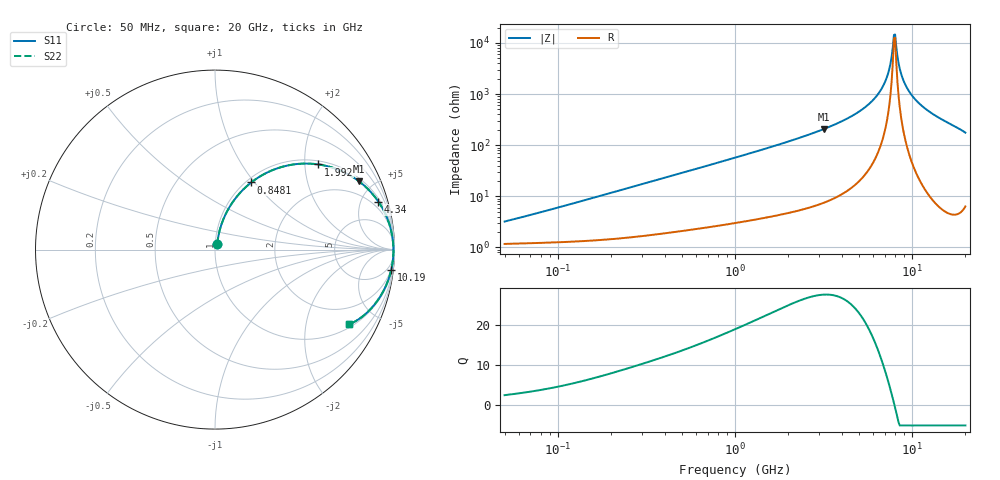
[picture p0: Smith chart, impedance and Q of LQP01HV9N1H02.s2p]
!Murata Part Number: LQP01HV9N1H02
!These Parameters are Measured in Series Mode Connection
!  o--[Z]--o
!Port1  Port2
!  o-------o
!Freq. Start=50[MHz] Stop=20[GHz], 401[Steps]
# Hz S RI R 50
!Freq.(Hz) S11(Real) S11(Imag) S21(Real) S21(Imag) S12(Real) S12(Imag) S22(Real) S22(Imag)
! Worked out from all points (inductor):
!   401 points, 50 MHz to 20 GHz, reference 50 ohm
!   read as one part in series: L = 9.43 nH near 60.75 MHz
!   highest Q = 27.6 at 3.169 GHz (marker M1), where L = 10.4 nH
!   self-resonance near 7.902 GHz
!   S11 on the Smith chart (normalised r, x): 50 MHz: 1.02, +0.06; 848.1 MHz: 1.05, +0.96; 1.992 GHz: 1.09, +2.35; 4.34 GHz: 1.26, +6.74; 10.19 GHz: 2, -17; 20 GHz: 1.13, -3.52
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5e7  0.0125 0.0292  0.9875 -0.0292  0.9875 -0.0292  0.0125 0.0292
1.364002e8  0.0192 0.0774  0.9808 -0.0774  0.9808 -0.0774  0.0192 0.0774
3.721004e8  0.0595 0.1977  0.9405 -0.1977  0.9405 -0.1977  0.0595 0.1977
8.480927e8  0.2023 0.3744  0.7977 -0.3744  0.7977 -0.3744  0.2023 0.3744
1e9  0.256 0.4109  0.744 -0.4109  0.744 -0.4109  0.256 0.4109
1.99176e9  0.5766 0.4745  0.4234 -0.4745  0.4234 -0.4745  0.5766 0.4745
2.728004e9  0.7352 0.4232  0.2648 -0.4232  0.2648 -0.4232  0.7352 0.4232
3.168813e9  0.8016 0.3811  0.1984 -0.3811  0.1984 -0.3811  0.8016 0.3811
4.34015e9  0.9106 0.2667  0.0894 -0.2667  0.0894 -0.2667  0.9106 0.2667
5.352748e9  0.958 0.1783  0.042 -0.1783  0.042 -0.1783  0.958 0.1783
6.217679e9  0.9797 0.1121  0.0203 -0.1121  0.0203 -0.1121  0.9797 0.1121
6.905011e9  0.989 0.0649  0.011 -0.0649  0.011 -0.0649  0.989 0.0649
7.442007e9  0.9928 0.0309  0.00723 -0.0309  0.00723 -0.0309  0.9928 0.0309
7.784049e9  0.9939 0.0104  0.00614 -0.0104  0.00614 -0.0104  0.9939 0.0104
8.020766e9  0.9941 -0.00335  0.0059 0.00335  0.0059 0.00335  0.9941 -0.00335
8.141811e9  0.9941 -0.0102  0.00593 0.0102  0.00593 0.0102  0.9941 -0.0102
8.516016e9  0.9934 -0.0309  0.00659 0.0309  0.00659 0.0309  0.9934 -0.0309
8.774992e9  0.9925 -0.0446  0.00753 0.0446  0.00753 0.0446  0.9925 -0.0446
9.316812e9  0.9894 -0.0723  0.0106 0.0723  0.0106 0.0723  0.9894 -0.0723
1.019291e10  0.9817 -0.1138  0.0183 0.1138  0.0183 0.1138  0.9817 -0.1138
1.314879e10  0.9381 -0.2311  0.0619 0.2311  0.0619 0.2311  0.9381 -0.2311
2e10  0.7485 -0.4162  0.2515 0.4162  0.2515 0.4162  0.7485 -0.4162
